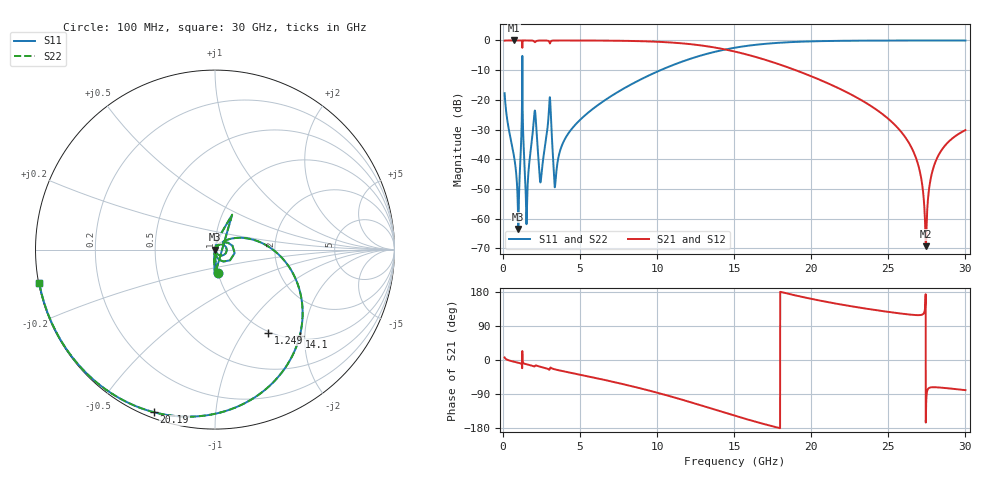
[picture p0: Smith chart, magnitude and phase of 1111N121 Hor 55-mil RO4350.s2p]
# GHz S MA R 50
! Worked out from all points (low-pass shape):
!   3201 points, 100 MHz to 30 GHz, reference 50 ohm
!   highest |S21| = -0.01 dB at 688.7 MHz (marker M1); lowest = -69.3 dB at 27.43 GHz (marker M2)
!   |S21| within 3 dB of the highest: start of sweep to 14.38 GHz
!   lowest |S11| = -63.5 dB at 987.7 MHz (marker M3), VSWR 1.00, Z = 50.1 - j0.0212 ohm
!   |S11| at or under -10 dB: start of sweep to 1.244 GHz; 1.253 GHz to 10.22 GHz (8.969 GHz wide, 156 % of centre)
!   |S22| runs from -63.5 to 0.0 dB; largest |S21 - S12| = 0
!   S11 on the Smith chart (normalised r, x): 100 MHz: 1.00, -0.26; 1.249 GHz: 0.99, -1.31; 14.1 GHz: 1.06, -1.88; 20.19 GHz: 0.02, -0.69; 30 GHz: 0.00, -0.09
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0.1  0.1295 -83.2  0.9913 6.7  0.9913 6.7  0.1295 -83.2
0.6886562  0.01208 -92.0  0.9993 -4.4  0.9993 -4.4  0.01208 -92.0
0.9876563  0.0006689 -18.5  0.9992 -7.3  0.9992 -7.3  0.0006689 -18.5
1.249281  0.5493 -57.3  0.7528 23.6  0.7528 23.6  0.5493 -57.3
1.548281  0.001682 47.2  0.9989 -11.5  0.9989 -11.5  0.001682 47.2
2.024812  0.05661 26.2  0.9578 -17.2  0.9578 -17.2  0.05661 26.2
2.454625  0.004427 16.1  0.9961 -18.2  0.9961 -18.2  0.004427 16.1
3.024594  0.1072 1.8  0.9028 -25.0  0.9028 -25.0  0.1072 1.8
3.407688  0.004392 24.3  0.9967 -25.1  0.9967 -25.1  0.004392 24.3
3.921594  0.01968 55.4  0.9977 -29.7  0.9977 -29.7  0.01968 55.4
5.089563  0.04855 48.6  0.9967 -39.6  0.9967 -39.6  0.04855 48.6
10.06978  0.3039 2.5  0.949 -87.0  0.949 -87.0  0.3039 2.5
14.09694  0.6756 -45.7  0.7312 -135.4  0.7312 -135.4  0.6756 -45.7
15.05  0.755 -57.5  0.649 -147.2  0.649 -147.2  0.755 -57.5
20.03956  0.9655 -109.3  0.247 161.1  0.247 161.1  0.9655 -109.3
20.18906  0.9677 -110.5  0.2381 159.8  0.2381 159.8  0.9677 -110.5
25.01978  0.9959 -143.9  0.04739 126.8  0.04739 126.8  0.9959 -143.9
26.73903  0.997 -153.3  0.01147 118.7  0.01147 118.7  0.997 -153.3
27.43047  0.997 -156.9  0.0003443 -165.0  0.0003443 -165.0  0.997 -156.9
27.76684  0.997 -158.6  0.004979 -72.2  0.004979 -72.2  0.997 -158.6
28.15928  0.997 -160.5  0.01042 -72.1  0.01042 -72.1  0.997 -160.5
30  0.9965 -169.2  0.03093 -79.5  0.03093 -79.5  0.9965 -169.2
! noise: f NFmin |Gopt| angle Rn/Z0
0.1  0.0006717  0.7366  1.095  0.0005098
3.417  0.01336  0.5916  24.99  0.005733
6.743  0.01553  0.4093  45.47  0.00374
10.06  0.02329  0.4352  62.41  0.005268
13.39  0.03536  0.5211  78.25  0.008293
16.7  0.05769  0.6525  95.8  0.01497
20.03  0.1086  0.7957  115.4  0.03237
23.35  0.2671  0.9113  135.1  0.09812
26.67  1.992  0.9872  153.1  1.999
30  0.8424  0.9694  169.1  0.05814
